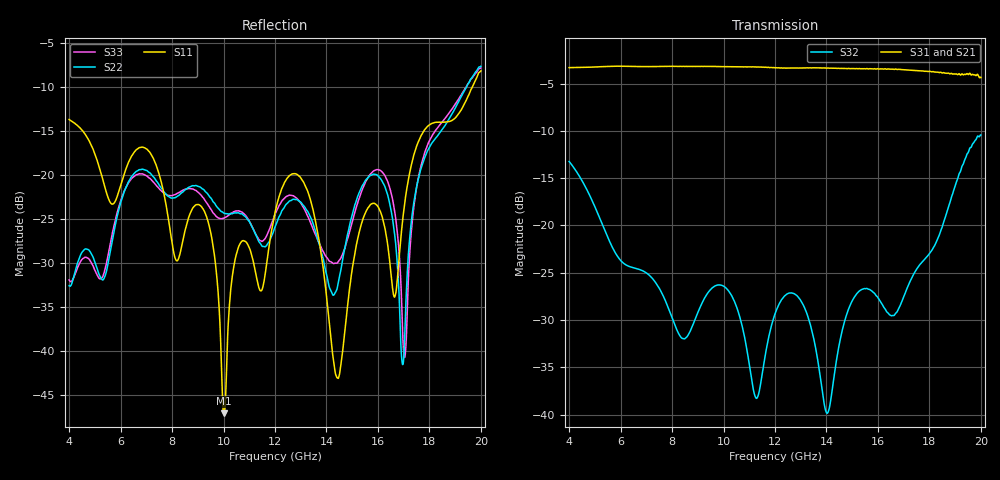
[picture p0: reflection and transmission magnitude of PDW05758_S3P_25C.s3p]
!Power divider measured mounted on 10mil RO4350 with coaxial edge launch connectors.  Coaxial connectors have been gated out.  Unused port was externally terminated
!with coaxial termination.  Measurement reference plane placed at the part edge.  The loss of the test board and connectors has been removed.
!This s3p file was manually constructed using three s2p files.  Symmetry was assumed (i.e. Sij = Sji)
!Port one = common port
!Port two = output port
!Port two = output port
# GHz S MA R 50
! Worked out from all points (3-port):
!   1601 points, 4 GHz to 20 GHz, reference 50 ohm
!   strongest paths, dB at 4 GHz, 8 GHz, 12 GHz, 16 GHz, 20 GHz:
!     S31: -3.3, -3.2, -3.3, -3.4, -4.4
!     S21: -3.3, -3.2, -3.3, -3.4, -4.4
!     S32: -13.2, -29.7, -29.4, -27.6, -10.4
!   lowest |S11| = -47.1 dB at 10.02 GHz (marker M1), VSWR 1.01, Z = 50 + j0.44 ohm
!   |S11| at or under -10 dB: start of sweep to 19.66 GHz
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4  0.2069 99.4  0.6839 -126.1  0.683 -125.5
   0.6839 -126.1  0.02343 89.2  0.218 -147.2
   0.683 -125.5  0.218 -147.2  0.02528 86.1
9.22  0.06359 32.7  0.6924 53.7  0.6926 54.9
      0.6924 53.7  0.08274 15.8  0.04021 -161.9
      0.6926 54.9  0.04021 -161.9  0.07401 17.3
10.02  0.004402 92.6  0.6906 24.1  0.6906 25.3
       0.6906 24.1  0.06068 47.5  0.04756 167.7
       0.6906 25.3  0.04756 167.7  0.05686 59.5
12  0.06109 -119.4  0.6817 -52.0  0.6817 -50.5
    0.6817 -52.0  0.05062 -37.9  0.03406 -161.5
    0.6817 -50.5  0.03406 -161.5  0.05969 -46.9
13.25  0.08222 -153.8  0.6814 -102.1  0.6814 -100.4
       0.6814 -102.1  0.06256 -66.2  0.03388 138.3
       0.6814 -100.4  0.03388 138.3  0.05914 -67.5
14.43  0.00702 160.3  0.6772 -152.3  0.6769 -150.4
       0.6772 -152.3  0.02319 44.2  0.02093 -152.0
       0.6769 -150.4  0.02093 -152.0  0.0317 28.3
16.04  0.06445 133.0  0.6706 135.3  0.6711 137.3
       0.6706 135.3  0.09748 91.5  0.04058 158.1
       0.6711 137.3  0.04058 158.1  0.1069 96.6
16.96  0.05532 -115.8  0.6667 91.3  0.6665 93.4
       0.6667 91.3  0.008332 -14.8  0.04061 -178.7
       0.6665 93.4  0.04061 -178.7  0.01268 44.6
17.65  0.1642 -131.6  0.657 57.2  0.6564 59.5
       0.657 57.2  0.1059 -130.9  0.06251 177.4
       0.6564 59.5  0.06251 177.4  0.1092 -129.3
20  0.3912 100.7  0.6043 -62.7  0.6054 -59.6
    0.6043 -62.7  0.4162 92.5  0.3007 120.6
    0.6054 -59.6  0.3007 120.6  0.4065 93.6
